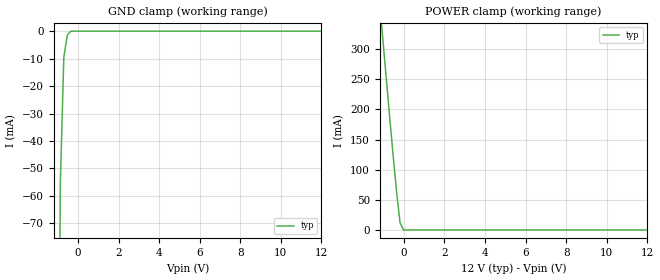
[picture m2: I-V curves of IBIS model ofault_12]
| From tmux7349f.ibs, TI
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| ofault_12
[Model]   ofault_12
Model_type   Input
Vinl = 0.8
Vinh = 1.3
|   typ   min   max
C_comp   2.533030e-12   NA   NA
[Voltage Range]   12   NA   NA
[Temperature Range]   27   NA   NA
[Power Clamp Reference]   12   NA   NA
[GND Clamp Reference]   0   NA   NA
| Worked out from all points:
|   GND clamp passes 1 mA (typ) near -0.48 V on its own axis
|   POWER clamp passes 1 mA (typ) near -0.03 V on its own axis
[GND Clamp]
|   Voltage   I(typ)   I(min)   I(max)
-5V       -36.55A    NA         NA
-1.051V   -258.3mA   NA         NA
-878.8mV  -55.69mA   NA         NA
-707.1mV  -9.535mA   NA         NA
-535.4mV  -1.483mA   NA         NA
-363.6mV  -33.47uA   NA         NA
12V       24.03uA    NA         NA
[POWER Clamp]
|   Voltage   I(typ)   I(min)   I(max)
-5V       1.876A     NA         NA
-1.222V   386.5mA    NA         NA
-1.05V    320mA      NA         NA
-707.1mV  188.5mA    NA         NA
-535.4mV  124.4mA    NA         NA
-363.6mV  62.94mA    NA         NA
-191.9mV  11.93mA    NA         NA
-20.2mV   52.31uA    NA         NA
12V       0A         NA         NA
